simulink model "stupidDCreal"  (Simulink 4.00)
settings: Solver=ode45  SolverMode=SingleTasking  StartTime=0.0  StopTime=100  RelTol=1e-3  AbsTol=1e-6
PostLoadFcn:
  | stupidDCpostloadfcn
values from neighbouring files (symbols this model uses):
  Ts = 0.01    [pidDCpostloadfcn.m]    (also in stupidDCpostloadfcn.m = 0.1)
undefined symbols (not defined in the file or in its folder): conv, polyc2d, polyval
libraries: adaptlib x2

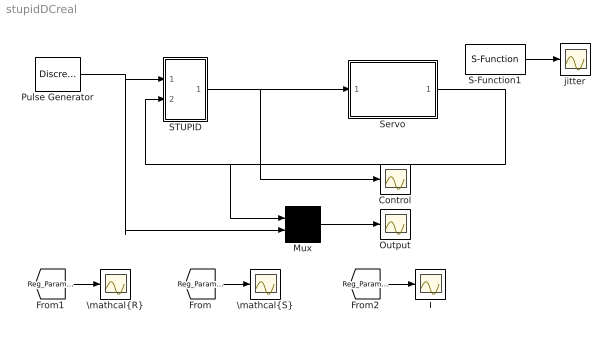
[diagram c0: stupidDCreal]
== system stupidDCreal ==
  Control : Scope
  Mux : Mux  Inputs=2
  Output : Scope
  Pulse Generator : DiscretePulseGenerator  PulseType=Time-based  Amplitude=2  Period=10  PulseWidth=50  PhaseDelay=0  SampleTime=1
  S-Function1 : S-Function  FunctionName=timer  Parameters=Ts  PortCounts=[]  SFunctionModules=''
  STUPID : Subsystem  mask{wo=5, zeta=1, theta0=[0.3;-0.1;2; -1], P0=100*diag([1 1 1 1]), lambda=, a_o=, h=Ts, d0=, um=10}
      mask prompts: wo "w_o (closed loop bandwidth)"; zeta "Closed loop damping"; theta0 "Initial estimate"; P0 "Initial covariance matrix"; lambda "Forgeting factor"; a_o "Observer pole"; h "Sampling time"; d0 "d0 (prediction horizon)"; um "Maximum control signal"
      mask help: DSTR with integral term.
  Servo : Subsystem
  T : Scope
  "\\mathcal{R}" : Scope
  "\\mathcal{S}" : Scope
  jitter : Scope
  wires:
  Mux/1 -> Output/1
  Pulse Generator/1 -> Mux/2, STUPID/1(u_c)
  STUPID/1(u) -> Control/1, Servo/1(u)
  Servo/1(p_2) -> Mux/1, STUPID/2(y)
  [Reg_ParametersStilde] -> "\\mathcal{S}"/1
  [Reg_ParametersRtilde] -> "\\mathcal{R}"/1
  [Reg_ParametersT] -> T/1
  S-Function1/1 -> jitter/1

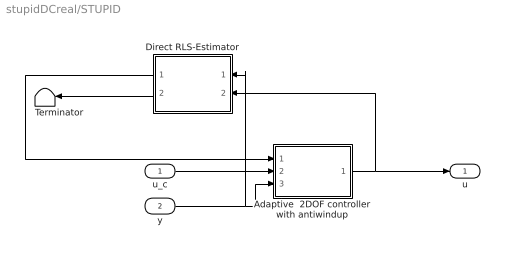
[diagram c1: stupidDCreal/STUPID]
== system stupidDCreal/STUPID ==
  u_c : Inport  Port=1  LatchInput=off
  y : Inport  Port=2  LatchInput=off
  Adaptive  2DOF controller with antiwindup : Subsystem  AncestorBlock=|  mask{n_r=2, ulim=um, A_m=polyc2d([1 2*zeta*wo wo^2],h), A_o=[1 -a_o], A_ow=polyc2d([1 2*0.7*7 7^2],h), h=h}
      | adaptlib/Adaptive 
      | 2DOF controller
      | with antiwindup
      mask prompts: n_r "n_r (degree of R, S and T)"; ulim "Maximum control signal"; A_o "A_o (Observer polynomial)"; A_ow "A_ow (Anti windup polynomial)"; h "Sampling period"
      mask help: A two-degree-of-freedom linear controller with control signal saturation and anti windup. A_o(q)v(k)=T(q)u_c(k)-S(q)y(k)-(A_o(q)-R(q))u(t) u(k)=f(v(k))
  Direct RLS-Estimator : Subsystem  Orientation=left  Priority=1  AncestorBlock=adaptlib/Direct RLS-Estimator  mask{n_r=1, theta_0=theta0, P_0=P0, lambda=lambda, A_m=polyc2d([1 2*zeta*wo wo^2],h), A_o=[1 -a_o], d0=d0, h=h}
      mask prompts: n_r "n_r (degree of estimated R, S )"; theta_0 "Initial estimate"; P_0 "Initial covariance matrix"; h "Sampling period"
  Terminator : Terminator
  u : Outport  Port=1
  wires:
  Adaptive  2DOF controller with antiwindup/1(u) -> u/1, Direct RLS-Estimator/2(u)
  y/1 -> Direct RLS-Estimator/1(y), Adaptive  2DOF controller with antiwindup/3(y)
  u_c/1 -> Adaptive  2DOF controller with antiwindup/2(u_c)
  Direct RLS-Estimator/1("[R,S,T]") -> Adaptive  2DOF controller with antiwindup/1("[R,S,T]")
  Direct RLS-Estimator/2(P) -> Terminator/1

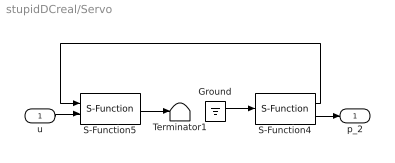
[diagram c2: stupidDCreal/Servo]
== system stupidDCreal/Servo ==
  u : Inport  Port=1  LatchInput=off
  Ground : Ground
  S-Function4 : S-Function  FunctionName=analogin  Parameters=Ts [0]  PortCounts=[]  SFunctionModules=''
  S-Function5 : S-Function  FunctionName=analogout  Parameters=Ts [0]  PortCounts=[]  SFunctionModules=''
  Terminator1 : Terminator
  p_2 : Outport  Port=1
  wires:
  u/1 -> S-Function5/2
  S-Function4/2 -> p_2/1
  S-Function4/1 -> S-Function5/1
  S-Function5/1 -> Terminator1/1
  Ground/1 -> S-Function4/1

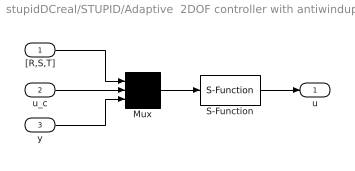
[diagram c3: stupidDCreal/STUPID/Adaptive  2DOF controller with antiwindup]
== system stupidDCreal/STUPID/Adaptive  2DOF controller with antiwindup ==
  "[R,S,T]" : Inport  Port=1  LatchInput=off
  u_c : Inport  Port=2  LatchInput=off
  y : Inport  Port=3  LatchInput=off
  Mux : Mux  Inputs=3
  S-Function : S-Function  FunctionName=rstdirint  Parameters=2,h,A_o,A_ow,A_m,ulim  PortCounts=[]  SFunctionModules=''
  u : Outport  Port=1  InitialOutput=0
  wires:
  u_c/1 -> Mux/2
  S-Function/1 -> u/1
  Mux/1 -> S-Function/1
  y/1 -> Mux/3
  "[R,S,T]"/1 -> Mux/1

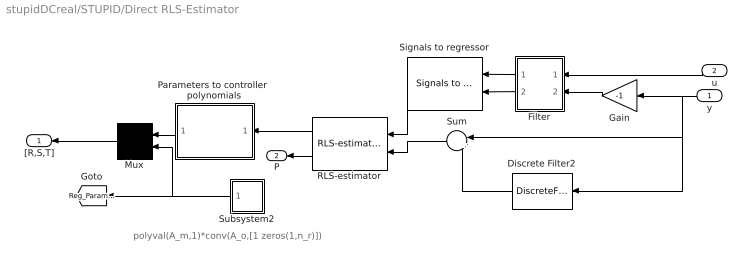
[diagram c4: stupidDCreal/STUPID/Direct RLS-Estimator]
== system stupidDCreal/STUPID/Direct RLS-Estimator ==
  note: polyval(A_m,1)*conv(A_o,[1 zeros(1,n_r)])
  y : Inport  Orientation=left  Port=1  LatchInput=off
  u : Inport  Orientation=left  Port=2  LatchInput=off
  Discrete Filter2 : DiscreteFilter  Orientation=left  Numerator=[zeros(1,d0) 1]*polyval(A_m,1)*polyval(A_o,1)  Denominator=conv(A_m,A_o)  SampleTime=h  Realization=auto
  Filter : Subsystem  Orientation=left  mask{A_m=A_m, A_o=A_o, d0=d0, h=h}
  Gain : Gain  Orientation=left  Gain=-1  Multiplication=Element-wise(K.*u)  SaturateOnIntegerOverflow=on
  Mux : Mux  Orientation=left  Inputs=2
  Parameters to controller  polynomials : Subsystem  Orientation=left  AncestorBlock="adaptlib/Parameters to controller  polynomials"  mask{n_r=n_r}
      mask prompts: n_r "n_r (degree of R, S )"
  RLS-estimator : adaptlib/RLS-estimator  Orientation=left  n=2*(n_r+1)  theta_0=theta_0  P_0=P_0  lambda=lambda  h=h
  Signals to regressor : adaptlib/Signals to regressor  Orientation=left  m=n_r+1  n=n_r+1  h=h
  Subsystem2 : Subsystem  Orientation=left
  Sum : Sum  Orientation=left  Inputs=|+-  SaturateOnIntegerOverflow=on
  "[R,S,T]" : Outport  Orientation=left  Port=1  InitialOutput=0
  P : Outport  Orientation=left  Port=2  InitialOutput=0
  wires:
  Subsystem2/1(Out1) -> [Reg_ParametersT], Mux/2
  Discrete Filter2/1 -> Sum/2
  Sum/1 -> RLS-estimator/2
  Parameters to controller  polynomials/1("[R,S]") -> Mux/1
  RLS-estimator/1 -> Parameters to controller  polynomials/1(theta)
  RLS-estimator/2 -> P/1
  Signals to regressor/1 -> RLS-estimator/1
  Filter/2(y_f) -> Signals to regressor/2
  Filter/1(u_f) -> Signals to regressor/1
  y/1 -> Discrete Filter2/1, Sum/1, Gain/1
  u/1 -> Filter/1(u)
  Gain/1 -> Filter/2(y)
  Mux/1 -> "[R,S,T]"/1

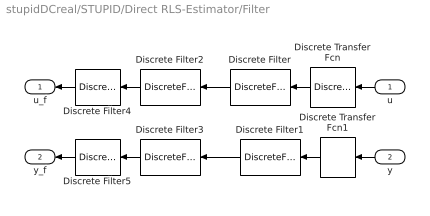
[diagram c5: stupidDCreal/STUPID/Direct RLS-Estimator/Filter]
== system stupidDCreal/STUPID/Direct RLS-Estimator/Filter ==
  u : Inport  Orientation=left  Port=1  LatchInput=off
  y : Inport  Orientation=left  Port=2  LatchInput=off
  Discrete Transfer Fcn : DiscreteTransferFcn  Orientation=left  Numerator=[1]  Denominator=[1 zeros(1,d0) ]  SampleTime=h  Realization=auto
  Discrete Transfer Fcn1 : DiscreteTransferFcn  Orientation=left  Numerator=[1]  Denominator=[1 zeros(1,d0) ]  SampleTime=h  Realization=auto
  Discrete Filter : DiscreteFilter  Orientation=left  Numerator=[1]  Denominator=A_o  SampleTime=h  Realization=auto
  Discrete Filter1 : DiscreteFilter  Orientation=left  Numerator=[1]  Denominator=A_o  SampleTime=h  Realization=auto
  Discrete Filter2 : DiscreteFilter  Orientation=left  Numerator=[1]  Denominator=A_m  SampleTime=h  Realization=auto
  Discrete Filter3 : DiscreteFilter  Orientation=left  Numerator=[1]  Denominator=A_m  SampleTime=h  Realization=auto
  Discrete Filter4 : DiscreteFilter  Orientation=left  Numerator=[1 -1]  Denominator=[1]  SampleTime=h  Realization=auto
  Discrete Filter5 : DiscreteFilter  Orientation=left  Numerator=[1 -1]  Denominator=[1 ]  SampleTime=h  Realization=auto
  u_f : Outport  Orientation=left  Port=1  InitialOutput=0
  y_f : Outport  Orientation=left  Port=2  InitialOutput=0
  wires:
  Discrete Filter5/1 -> y_f/1
  Discrete Filter4/1 -> u_f/1
  Discrete Transfer Fcn1/1 -> Discrete Filter1/1
  Discrete Transfer Fcn/1 -> Discrete Filter/1
  Discrete Filter1/1 -> Discrete Filter3/1
  Discrete Filter/1 -> Discrete Filter2/1
  y/1 -> Discrete Transfer Fcn1/1
  u/1 -> Discrete Transfer Fcn/1
  Discrete Filter3/1 -> Discrete Filter5/1
  Discrete Filter2/1 -> Discrete Filter4/1

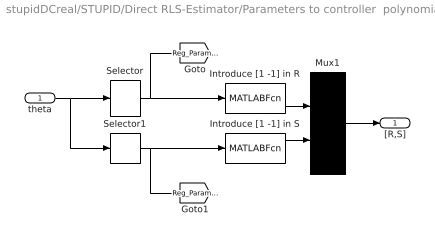
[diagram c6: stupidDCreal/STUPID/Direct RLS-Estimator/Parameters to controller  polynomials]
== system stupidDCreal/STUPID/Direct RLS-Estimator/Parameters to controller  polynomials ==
  theta : Inport  Port=1  LatchInput=off
  Introduce [1 -1] in R : MATLABFcn  MATLABFcn=conv(u,[1 -1])  OutputDimensions=3  OutputSignalType=auto  Output1D=on
  Introduce [1 -1] in S : MATLABFcn  MATLABFcn=conv(u,[1 -1])  OutputDimensions=3  OutputSignalType=auto  Output1D=on
  Mux1 : Mux  Inputs=2
  Selector : Selector  InputType=Vector  ElementSrc=Internal  Elements=[1 : n_r+1]  RowSrc=Internal  Rows=1  ColumnSrc=Internal  Columns=1  InputPortWidth=2*(n_r+1)
  Selector1 : Selector  InputType=Vector  ElementSrc=Internal  Elements="[n_r+2 :  2*(n_r+1)]"  RowSrc=Internal  Rows=1  ColumnSrc=Internal  Columns=1  InputPortWidth=2*(n_r+1)
  "[R,S]" : Outport  Port=1  InitialOutput=0
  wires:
  Introduce [1 -1] in S/1 -> Mux1/2
  Introduce [1 -1] in R/1 -> Mux1/1
  theta/1 -> Selector1/1, Selector/1
  Selector/1 -> [Reg_ParametersRtilde], Introduce [1 -1] in R/1
  Mux1/1 -> "[R,S]"/1
  Selector1/1 -> [Reg_ParametersStilde], Introduce [1 -1] in S/1

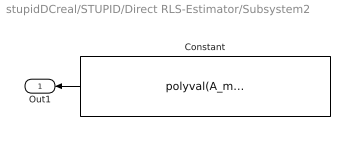
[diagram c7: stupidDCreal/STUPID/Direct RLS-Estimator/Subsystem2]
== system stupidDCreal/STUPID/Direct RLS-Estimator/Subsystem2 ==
  Constant : Constant  Orientation=left  Value=polyval(A_m,1)*conv(A_o,[1 zeros(1,n_r)])
  Out1 : Outport  Orientation=left  Port=1
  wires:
  Constant/1 -> Out1/1
